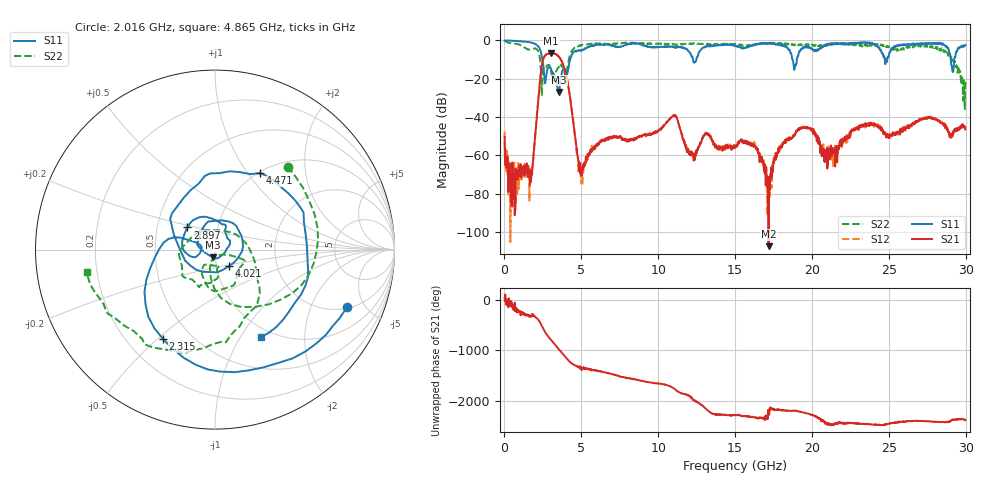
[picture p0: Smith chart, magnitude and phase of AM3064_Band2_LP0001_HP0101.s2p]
# Hz S DB R 50.0
!freq dBS11 angS11 dBS21 angS21 dBS12 angS12 dBS22 angS22
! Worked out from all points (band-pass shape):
!   1600 points, 10 MHz to 29.98 GHz, reference 50 ohm
!   highest |S21| = -6.60 dB at 3.046 GHz (marker M1); lowest = -107.5 dB at 17.18 GHz (marker M2)
!   |S21| within 3 dB of the highest: 2.536 GHz to 3.64 GHz (1.103 GHz wide, 35.7 % of centre)
!   lowest |S11| = -27.0 dB at 3.553 GHz (marker M3), VSWR 1.09, Z = 48.5 - j4.13 ohm
!   |S11| at or under -10 dB: 2.463 GHz to 4.273 GHz (1.811 GHz wide, 53.8 % of centre); 18.73 GHz to 19.02 GHz (287.9 MHz wide, 1.53 % of centre); 29.02 GHz to 29.25 GHz (229.9 MHz wide, 0.789 % of centre)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
!   |S22| runs from -35.9 to -0.2 dB; largest |S21 - S12| = 0.015
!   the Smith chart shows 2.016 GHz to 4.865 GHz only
!   S11 on the Smith chart (normalised r, x): 2.016 GHz: 2.08, -3.74; 2.315 GHz: 0.35, -0.52; 2.897 GHz: 0.71, +0.18; 4.021 GHz: 1.15, -0.21; 4.471 GHz: 1.01, +1.14; 4.865 GHz: 0.87, -1.23
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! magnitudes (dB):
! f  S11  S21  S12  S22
! 10 MHz  0.0  -50.4  -47.6  -0.2
! 816 MHz  -0.3  -71.1  -69.2  -1.9
! 1.716 GHz  -1.1  -71.2  -68.9  -4.6
! 2.016 GHz  -1.9  -48.4  -48.6  -4.2
! 2.315 GHz  -4.8  -21.0  -20.9  -10.0
! 2.897 GHz  -14.1  -6.9  -6.8  -12.7
! 3.046 GHz  -15.2  -6.6  -6.6  -17.0
! 3.553 GHz  -27.0  -8.8  -8.5  -13.2
! 4.021 GHz  -18.4  -18.5  -18.4  -17.7
! 4.471 GHz  -6.1  -42.1  -42.2  -4.4
! 4.865 GHz  -5.2  -67.9  -68.9  -2.8
! 5.015 GHz  -5.3  -70.7  -74.7  -2.6
! 10 GHz  -3.4  -47.4  -47.2  -1.7
! 15 GHz  -2.6  -56.0  -55.2  -1.8
! 16.28 GHz  -2.2  -55.2  -54.0  -2.3
! 17.18 GHz  -1.8  -107.5  -72.6  -1.6
! 18.21 GHz  -2.6  -53.0  -52.8  -1.7
! 19.99 GHz  -4.2  -46.5  -47.1  -2.1
! 20.95 GHz  -2.5  -57.3  -57.4  -2.2
! 25 GHz  -8.2  -50.8  -48.8  -3.1
! 28.56 GHz  -2.3  -44.4  -43.6  -5.0
! 29.98 GHz  -2.4  -46.6  -45.7  -21.7
